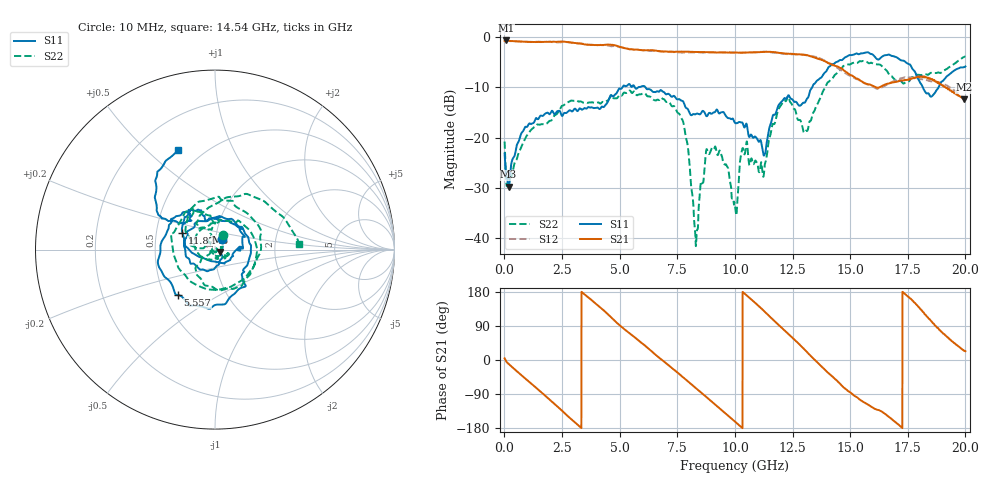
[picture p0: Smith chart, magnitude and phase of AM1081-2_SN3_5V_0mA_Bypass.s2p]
!Agilent Technologies,E8364B,MY43040894,A.07.50.67
!Agilent E8364B: A.07.50.67
!Date: Wednesday, June 23, 2021 08:06:22
!Correction: S11(Full 2 Port(1,2))
!S21(Full 2 Port(1,2))
!S12(Full 2 Port(1,2))
!S22(Full 2 Port(1,2))
!S2P File: Measurements: S11, S21, S12, S22:
# Hz S  dB  R 50
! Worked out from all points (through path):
!   3201 points, 10 MHz to 20 GHz, reference 50 ohm
!   highest |S21| = -0.64 dB at 72.47 MHz (marker M1); lowest = -12.4 dB at 19.95 GHz (marker M2)
!   group delay of S21, straight-line fit = 147 ps
!   lowest |S11| = -29.8 dB at 184.9 MHz (marker M3), VSWR 1.07, Z = 53.1 - j1.33 ohm
!   |S11| at or under -10 dB: start of sweep to 5.113 GHz; 6.125 GHz to 13.35 GHz (7.226 GHz wide, 74.2 % of centre); 18.15 GHz to 18.83 GHz (679 MHz wide, 3.67 % of centre)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
!   |S22| runs from -41.6 to -3.9 dB; largest |S21 - S12| = 0.031
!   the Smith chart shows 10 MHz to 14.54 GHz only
!   S11 on the Smith chart (normalised r, x): 10 MHz: 1.08, +0.12; 5.557 GHz: 0.59, -0.33; 11.87 GHz: 0.68, +0.14; 14.54 GHz: 0.37, +0.63
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1e7  -23.13 54.5  -0.74 4.2  -0.67 3.6  -20.76 61.8
7.246875e7  -27.31 13.3  -0.64 -3.0  -0.67 -3.0  -28.30 12.7
1.849125e8  -29.75 -22.5  -0.73 -10.4  -0.75 -10.3  -27.27 -34.2
1.771619e9  -15.20 172.8  -0.93 -94.3  -0.92 -94.8  -17.28 110.1
3.345831e9  -14.37 31.4  -1.26 179.9  -1.26 -179.6  -12.84 -47.9
5.557225e9  -9.72 -129.2  -2.43 64.4  -2.38 64.4  -11.06 77.1
6.675416e9  -10.83 149.8  -2.75 7.8  -2.76 8.5  -12.45 -38.3
7.731138e9  -12.68 109.3  -2.86 -44.5  -3.06 -44.2  -16.52 -136.9
8.312097e9  -15.26 96.0  -2.94 -74.5  -3.05 -73.7  -41.47 134.3
9.061722e9  -14.97 50.9  -3.01 -113.3  -2.97 -112.3  -22.22 -20.9
1.0005e10  -17.04 2.4  -3.05 -162.5  -3.02 -162.4  -33.66 -162.8
1.042354e10  -17.94 -1.2  -3.07 175.2  -3.03 175.3  -23.28 111.5
1.127312e10  -23.47 -102.3  -2.91 128.7  -2.89 128.6  -26.53 121.6
1.187282e10  -13.75 152.4  -3.08 93.7  -3.20 94.1  -14.50 149.2
1.334083e10  -10.10 148.3  -3.86 7.9  -3.77 8.5  -15.91 125.5
1.454023e10  -4.58 110.5  -6.03 -61.4  -6.39 -63.0  -6.59 3.8
1.561469e10  -3.10 35.9  -9.12 -112.2  -9.13 -111.8  -4.74 -68.9
1.667042e10  -3.44 -5.1  -9.22 -149.5  -9.25 -146.3  -7.33 -148.5
1.756997e10  -5.38 -39.9  -8.33 164.4  -7.96 161.4  -8.70 80.7
1.853198e10  -11.79 -150.6  -8.39 101.7  -8.78 104.5  -7.10 -8.7
1.995002e10  -5.95 96.8  -12.38 24.4  -12.22 21.7  -3.88 -167.0
2e10  -5.81 94.1  -12.30 23.1  -12.24 20.0  -3.89 -169.7
